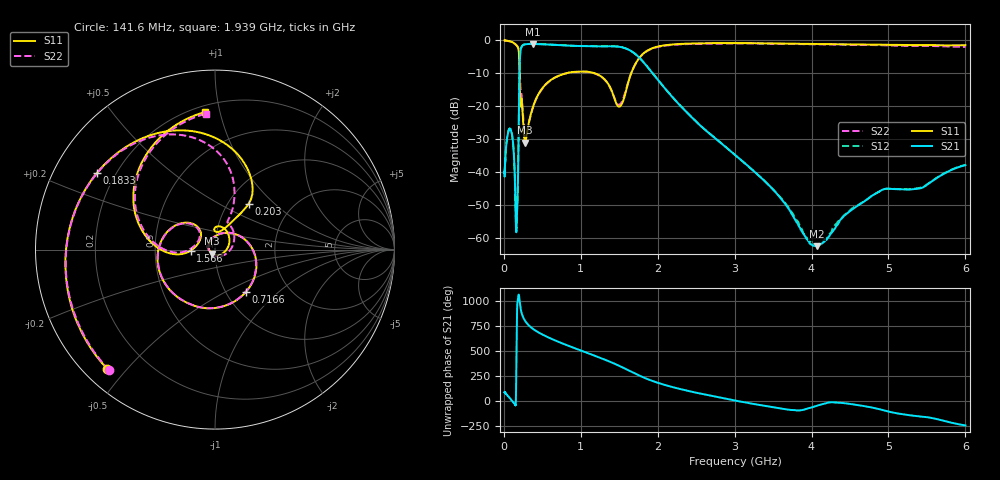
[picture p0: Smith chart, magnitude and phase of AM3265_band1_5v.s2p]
!Agilent Technologies,E8364B,MY43040894,A.07.50.67
!Agilent E8364B: A.07.50.67
!Date: Friday, May 09, 2025 07:15:52
!Correction: S11(Full 2 Port(1,2))
!S21(Full 2 Port(1,2))
!S12(Full 2 Port(1,2))
!S22(Full 2 Port(1,2))
!S2P File: Measurements: S11, S21, S12, S22:Log Frequency Sweep
# Hz S  dB  R 50
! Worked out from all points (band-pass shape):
!   3201 points, 10 MHz to 6 GHz, reference 50 ohm
!   highest |S21| = -1.06 dB at 375 MHz (marker M1); lowest = -62.5 dB at 4.071 GHz (marker M2)
!   |S21| within 3 dB of the highest: 212.6 MHz to 1.706 GHz (1.493 GHz wide, 156 % of centre)
!   lowest |S11| = -31.0 dB at 277.3 MHz (marker M3), VSWR 1.06, Z = 48.3 - j2.14 ohm
!   |S11| at or under -10 dB: 203 MHz to 804.9 MHz (601.9 MHz wide, 119 % of centre); 1.185 GHz to 1.655 GHz (470.1 MHz wide, 33.1 % of centre)
!   |S22| runs from -29.8 to 0.0 dB; largest |S21 - S12| = 0.0078
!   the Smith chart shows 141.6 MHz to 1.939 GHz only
!   S11 on the Smith chart (normalised r, x): 141.6 MHz: 0.07, -0.44; 183.3 MHz: 0.13, +0.29; 203 MHz: 1.24, +0.71; 716.6 MHz: 1.24, -0.64; 1.566 GHz: 0.76, -0.01; 1.939 GHz: 0.24, +0.90
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1e7  0.00 -7.8  -41.36 88.6  -40.58 37.2  -0.09 -7.7
2.908064e7  -0.06 -22.5  -32.43 68.3  -32.30 68.1  -0.06 -22.5
8.439949e7  -0.27 -68.7  -26.93 20.6  -26.86 19.8  -0.30 -68.8
1.416434e8  -0.96 -132.2  -40.71 -32.6  -40.32 -35.3  -0.98 -131.5
1.609754e8  -1.37 -162.6  -58.17 -115.9  -57.33 -177.6  -1.37 -160.8
1.833119e8  -2.11 146.8  -42.97 -59.6  -43.47 -58.6  -2.04 152.1
2.029866e8  -9.94 53.7  -10.70 -63.4  -10.66 -63.4  -7.07 78.7
2.44949e8  -22.29 14.0  -1.50 125.5  -1.47 125.4  -21.06 2.3
2.772696e8  -31.04 -127.9  -1.17 77.0  -1.13 76.9  -29.75 -122.6
3.749698e8  -20.43 69.3  -1.06 0.5  -1.02 0.5  -20.70 72.4
7.123273e8  -10.75 -52.4  -1.40 -131.9  -1.36 -131.9  -10.76 -52.8
7.166121e8  -10.70 -53.6  -1.40 -133.3  -1.37 -133.3  -10.72 -54.0
1.169463e9  -9.88 -175.1  -1.79 93.2  -1.76 93.2  -9.95 -176.0
1.565812e9  -17.29 -177.4  -2.28 -35.4  -2.26 -35.4  -16.73 -179.5
1.939251e9  -2.28 94.0  -10.13 -164.6  -10.11 -164.6  -2.39 93.9
2.067357e9  -1.55 62.8  -13.83 163.2  -13.81 163.3  -1.68 63.1
2.455151e9  -0.91 -11.0  -23.65 87.7  -23.63 87.7  -1.05 -10.4
2.96862e9  -0.79 -90.1  -34.07 7.1  -34.09 6.8  -0.90 -90.3
3.525473e9  -0.91 -167.4  -46.00 -69.4  -45.91 -70.0  -1.01 -169.3
4.071232e9  -1.08 121.1  -62.55 -49.9  -61.96 -54.9  -1.18 118.7
5.012054e9  -1.36 3.1  -45.09 -110.8  -45.10 -109.7  -1.54 3.6
6e9  -1.44 -115.2  -37.93 112.7  -37.80 112.1  -1.95 -110.9
